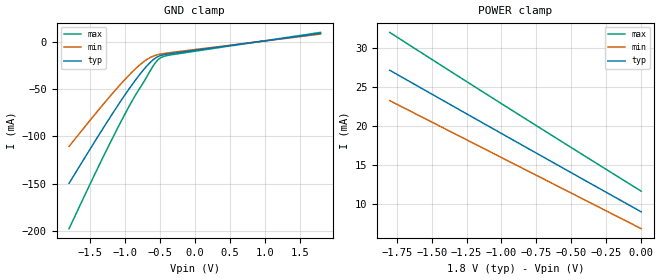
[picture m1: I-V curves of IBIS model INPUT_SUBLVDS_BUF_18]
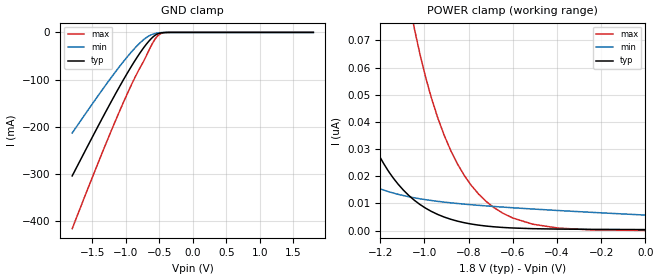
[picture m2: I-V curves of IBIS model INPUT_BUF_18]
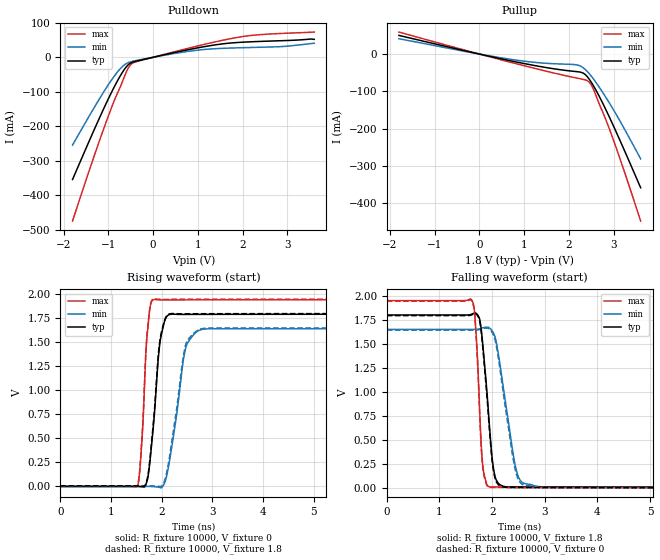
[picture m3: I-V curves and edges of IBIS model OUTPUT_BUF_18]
| TEXAS INSTRUMENTS INCORPORATED
| Digital Light Processing Group
| IBIS Model of d9696kx2sv
| P46_AUTO
| This device can be powered at the following Vccs:
|  1.8 volt Vcc
| This file provides unique models under the [Model Selector] for each Vcc.
| For operation at a specific Vcc, select the appropriate model after each
| [Model Selector] keyword.
[IBIS Ver]   3.2
[Comment char]  |_char
[File Name]   p46_auto_d9696kx2sv.ibs
[File Rev]   2.0 | f_die
[Date]   May 5, 2022
[Source]   Data created from TI-SPICE simulations at TI-DLP.
[Notes]   The following is an IBIS list for the 0.46 AUTO .
##notes##|
[Disclaimer] Property of Texas Instruments Incorporated.  Unauthorized
   reproduction and/or distribution is strictly prohibited.
   This product is protected under copyright law.
   Created  2022, (C) Copyright  2022, Texas Instruments
   Incorporated, All Rights Reserved
   UNLESS THERE IS A SIGNED, WRITTEN AGREEMENT TO THE
   CONTRARY, TEXAS INSTRUMENTS (TI) IS PROVIDING THE IBIS
   MODELS  AND WITHOUT ANY WARRANTY, EXPRESSED OR
   IMPLIED.  TI assumes no liability for:
   1) the accuracy of the IBIS models provided to your
   company;
   2) the proper functioning of these IBIS Models in your
   design or for any resulting applications; or
   3) infringement of patents, copyrights or intellectual
   property rights resulting from your use of these IBIS
   models.
   TI provides IBIS Models as a service to our customers.
   You and your company shall not distribute, sell or give
   these models to anyone else without prior written
   permission from TI.
   TI reserves the right to make changes to our products or
   to discontinue any semiconductor product or service
   without notice, and advises our customers to obtain the
   latest version of relevant information to verify, before
   placing orders, that the information being relied on is
   current.
   Please be aware that your receipt and use of the IBIS
   information provided shall serve as acceptance of these
   terms and conditions.  If you do not accept these terms,
   you should return or destroy the IBIS models and any
   other accompanying information immediately.
| Component P46_AUTO
[Component]   P46_AUTO
[Manufacturer]   Texas Instruments, Inc.
[Package]
|   typ   min   max
R_pkg   1.216   0.4680   2.140
L_pkg   6.179E-09   3.200E-09   1.320E-08
C_pkg   2.358E-12   1.500E-12   5.200E-12
|   Signal RLC
[Pin]   signal_name   model_name   R_pin   L_pin   C_pin
 A3   D_AN<0>   INPUT_SUB_LVDS_BUF   1.478   7.3E-09   2.5E-12
 B1   D_AN<1>   INPUT_SUB_LVDS_BUF   1.455   7.4E-09   2.5E-12
 C2   D_AN<2>   INPUT_SUB_LVDS_BUF   1.501   8.2E-09   2.5E-12
 F2   D_AN<3>   INPUT_SUB_LVDS_BUF   0.960   5.4E-09   2.0E-12
 H2   D_AN<4>   INPUT_SUB_LVDS_BUF   1.377   6.8E-09   2.4E-12
 K1   D_AN<5>   INPUT_SUB_LVDS_BUF   1.312   7.1E-09   2.3E-12
 K4   D_AN<6>   INPUT_SUB_LVDS_BUF   0.938   6.1E-09   2.0E-12
 K6   D_AN<7>   INPUT_SUB_LVDS_BUF   1.492   7.2E-09   2.5E-12
 A2   D_AP<0>   INPUT_SUB_LVDS_BUF   1.422   6.3E-09   2.4E-12
 C1   D_AP<1>   INPUT_SUB_LVDS_BUF   1.407   6.4E-09   2.4E-12
 D2   D_AP<2>   INPUT_SUB_LVDS_BUF   1.445   6.5E-09   2.4E-12
 E2   D_AP<3>   INPUT_SUB_LVDS_BUF   0.860   4.7E-09   2.0E-12
 G2   D_AP<4>   INPUT_SUB_LVDS_BUF   1.321   5.9E-09   2.3E-12
 K2   D_AP<5>   INPUT_SUB_LVDS_BUF   1.256   5.9E-09   2.3E-12
 K3   D_AP<6>   INPUT_SUB_LVDS_BUF   0.882   4.7E-09   2.0E-12
 K5   D_AP<7>   INPUT_SUB_LVDS_BUF   1.404   6.4E-09   2.4E-12
A22   D_BN<0>   INPUT_SUB_LVDS_BUF   1.504   6.8E-09   2.5E-12
B24   D_BN<1>   INPUT_SUB_LVDS_BUF   1.477   6.3E-09   2.5E-12
D23   D_BN<2>   INPUT_SUB_LVDS_BUF   1.154   5.3E-09   2.2E-12
F23   D_BN<3>   INPUT_SUB_LVDS_BUF   0.922   4.4E-09   1.9E-12
H23   D_BN<4>   INPUT_SUB_LVDS_BUF   1.302   6.0E-09   2.3E-12
K24   D_BN<5>   INPUT_SUB_LVDS_BUF   1.342   6.2E-09   2.4E-12
K21   D_BN<6>   INPUT_SUB_LVDS_BUF   0.894   4.9E-09   2.0E-12
K19   D_BN<7>   INPUT_SUB_LVDS_BUF   1.390   6.0E-09   2.4E-12
A23   D_BP<0>   INPUT_SUB_LVDS_BUF   1.446   6.4E-09   2.5E-12
C24   D_BP<1>   INPUT_SUB_LVDS_BUF   1.421   6.9E-09   2.4E-12
C23   D_BP<2>   INPUT_SUB_LVDS_BUF   1.096   5.8E-09   2.2E-12
E23   D_BP<3>   INPUT_SUB_LVDS_BUF   0.875   5.0E-09   1.9E-12
G23   D_BP<4>   INPUT_SUB_LVDS_BUF   1.246   5.7E-09   2.3E-12
K23   D_BP<5>   INPUT_SUB_LVDS_BUF   1.284   6.6E-09   2.3E-12
K22   D_BP<6>   INPUT_SUB_LVDS_BUF   0.839   5.1E-09   1.9E-12
K20   D_BP<7>   INPUT_SUB_LVDS_BUF   1.288   6.7E-09   2.4E-12
 J1   DCLK_AN   INPUT_SUB_LVDS_BUF   1.340   6.4E-09   2.4E-12
 H1   DCLK_AP   INPUT_SUB_LVDS_BUF   1.292   5.8E-09   2.3E-12
H24   DCLK_BN   INPUT_SUB_LVDS_BUF   1.187   5.3E-09   2.2E-12
J24   DCLK_BP   INPUT_SUB_LVDS_BUF   1.137   5.4E-09   2.2E-12
 E6   DMD_DEN_ARSTZ   INPUT_BUF   0.700   5.0E-09   2.4E-12
 C3   LS_CLK_N   INPUT_SUB_LVDS_BUF   0.468   3.2E-09   1.6E-12
 C4   LS_CLK_P   INPUT_SUB_LVDS_BUF   0.541   4.0E-09   1.5E-12
E19   LS_RDATA_A   OUTPUT_BUF   2.041   12.8E-09   5.0E-12
F19   LS_RDATA_B   OUTPUT_BUF   2.140   13.2E-09   5.2E-12
 C5   LS_WDATA_N   INPUT_SUB_LVDS_BUF   0.694   3.8E-09   1.8E-12
 C6   LS_WDATA_P   INPUT_SUB_LVDS_BUF   0.741   4.4E-09   1.8E-12
C18   MBRST<0>   NC
C17   MBRST<1>   NC
D18   MBRST<6>   NC
D17   MBRST<7>   NC
 F6   TEMP_N   NC
 G6   TEMP_P   NC
E18   TP0   NC
E17   TP1   NC
E16   TP2   NC
 A4   VBIAS   POWER
A21   VBIAS   POWER
A24   VSS   GND
 B2   VSS   GND
 B3   VOFFSET   POWER
 B4   VOFFSET   POWER
 B5   VSS   GND
 B6   VRESET   POWER
B19   VRESET   POWER
B20   VSS   GND
B21   VOFFSET   POWER
B22   VOFFSET   POWER
B23   VSS   GND
C19   VSS   GND
C20   VDD   POWER
C21   VSS   GND
C22   VSS   GND
 D3   VSS   GND
 D4   VDD   POWER
 D5   VSS   GND
 D6   VSS   GND
D19   VDD   POWER
D20   VSS   GND
D21   VDD   POWER
D22   VSS   GND
 E3   VDD   POWER
 E4   VSS   GND
 E5   VDDI   POWER
E20   VDDI   POWER
E21   VSS   GND
E22   VDD   POWER
 F3   VSS   GND
 F4   VDD   POWER
 F5   VDDI   POWER
F20   VDDI   POWER
F21   VSS   GND
F22   VSS   GND
 G3   VDD   POWER
 G4   VSS   GND
 G5   VDDI   POWER
G19   VSS   GND
G20   VDDI   POWER
G21   VDD   POWER
G22   VSS   GND
 H3   VSS   GND
 H4   VSS   GND
 H5   VDDI   POWER
 H6   VSS   GND
H19   VSS   GND
H20   VDDI   POWER
H21   VSS   GND
H22   VDD   POWER
 J2   VSS   GND
 J3   VDD   POWER
 J4   VOFFSET   POWER
 J5   VSS   GND
 J6   VDD   POWER
J19   VDD   POWER
J20   VSS   GND
J21   VOFFSET   POWER
J22   VSS   GND
J23   VSS   GND
| NOTE:  The [Diff Pin] section may get flagged by early versions of the
|   ibischk program
[Diff Pin]  inv_pin   vdiff   tdelay_typ
A2   A3   200mv   NA
C1   B1   200mv   NA
D2   C2   200mv   NA
E2   F2   200mv   NA
G2   H2   200mv   NA
K2   K1   200mv   NA
K3   K4   200mv   NA
K5   K6   200mv   NA
A23   A22   200mv   NA
C24   B24   200mv   NA
C23   D23   200mv   NA
E23   F23   200mv   NA
G23   H23   200mv   NA
K23   K24   200mv   NA
K22   K21   200mv   NA
K20   K19   200mv   NA
H1   J1   200mv   NA
J24   H24   200mv   NA
C4   C3   200mv   NA
C6   C5   200mv   NA
| Model INPUT_SUB_LVDS_BUF
[Model Selector]   INPUT_SUB_LVDS_BUF
INPUT_SUBLVDS_BUF_18   1.8 volt Vcc
| Model INPUT_BUF
[Model Selector]   INPUT_BUF
INPUT_BUF_18   1.8 volt Vcc
| Model OUTPUT_BUF
[Model Selector]   OUTPUT_BUF
OUTPUT_BUF_18   1.8 volt Vcc
| Models and submodels in the file (3): INPUT_SUBLVDS_BUF_18 (Input), INPUT_BUF_18 (Input), OUTPUT_BUF_18 (Output)
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[Model]   INPUT_SUBLVDS_BUF_18
Model_type  Input
Vinl=0.80
Vinh=1.00
| variable   typ   min   max
C_comp   0.69pF   0.66pF   0.72pF
[Temperature Range]   25   85   -40
[Voltage range]   1.8   1.65   1.95
[GND Clamp]
| INPUT_SUBLVDS_BUF_18
|   Voltage   I(typ)   I(min)   I(max)
-1.8V     -149.7mA   -110.7mA   -197.8mA
-1.29V    -88.84mA   -64.29mA   -118.6mA
-1.095V   -66.55mA   -47.56mA   -89.83mA
-930mV    -48.67mA   -34.42mA   -66.87mA
-790mV    -34.7mA    -24.56mA   -49.3mA
-680mV    -25.03mA   -18.39mA   -35.98mA
-580mV    -18.08mA   -14.73mA   -23.73mA
-510mV    -15.09mA   -13.26mA   -17.94mA
-450mV    -13.75mA   -12.43mA   -15.53mA
-355mV    -12.57mA   -11.45mA   -13.96mA
1.8V      8.993mA    8.203mA    9.976mA
[POWER Clamp]
| INPUT_SUBLVDS_BUF_18
|   Voltage   I(typ)   I(min)   I(max)
-1.8V     27.16mA    23.26mA    32.02mA
-1.37V    22.79mA    19.34mA    27.08mA
-920mV    18.24mA    15.23mA    21.97mA
-16.28fV  8.993mA    6.835mA    11.65mA
[Model]   INPUT_BUF_18
Model_type  Input
Vinl=0.54
Vinh=1.26
| variable   typ   min   max
C_comp   0.51pF   0.44pF   0.58pF
[Temperature Range]   25   85   -40
[Voltage range]   1.8   1.65   1.95
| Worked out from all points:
|   GND clamp passes 1 mA (typ) near -0.47 V on its own axis
[GND Clamp]
| INPUT_BUF_18
|   Voltage   I(typ)   I(min)   I(max)
-1.8V     -304mA     -213.1mA   -415.8mA
-1.52V    -227.4mA   -155.6mA   -314.4mA
-1.29V    -165.7mA   -109.6mA   -233.4mA
-1.095V   -115.3mA   -72.59mA   -167.6mA
-930mV    -75.06mA   -43.75mA   -115.2mA
-790mV    -43.93mA   -22.51mA   -75.55mA
-680mV    -22.72mA   -9.755mA   -45.56mA
-580mV    -7.998mA   -2.996mA   -17.96mA
-510mV    -2.379mA   -972.8uA   -5.564mA
-450mV    -592.5uA   -304.6uA   -1.296mA
-355mV    -35.15uA   -32.8uA    -61.22uA
1.8V      384pA      6.33nA     42.47pA
[POWER Clamp]
| INPUT_BUF_18
|   Voltage   I(typ)   I(min)   I(max)
-1.8V     438.6nA    109.4nA    1.836uA
-1.7V     293.4nA    73.99nA    1.296uA
-1.565V   164.4nA    44.27nA    784.1nA
-1.4V     75.97nA    25.31nA    401.7nA
-1.255V   36.21nA    17.25nA    210.8nA
-1.155V   20.97nA    14.17nA    130.5nA
-1.045V   11.14nA    12.07nA    74.21nA
-970mV    7.14nA     11.1nA     49.29nA
-880mV    4.163nA    10.23nA    29.33nA
-685mV    1.408nA    8.888nA    8.453nA
-395mV    567.5pA    7.406nA    949.3pA
-16.28fV  384pA      5.724nA    60.79pA
[Model]   OUTPUT_BUF_18
Model_type  Output
Vref =   0
Rref =   10000
Cref =   10p
Vmeas =   1.2
| variable   typ   min   max
C_comp   0.65pF   0.45pF   1.15pF
| C_pullup   0.66pF   0.45pF   1.15pF
| C_pulldown   0.63pF   0.50pF   1.03pF
[Temperature Range]   25   85   -40
[Voltage range]   1.8   1.65   1.95
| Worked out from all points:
|   slope of the pulldown table from 0 to 0.27 V, typ, clamps not added: 34.3 ohm
|   slope of the pullup table from 0 to 0.27 V, typ, clamps not added: 37.6 ohm
|   rising waveform, R_fixture 10000, V_fixture 0: 20-80 % time 164ps typ, 253ps min, 111ps max; typ from 0 V to 1.79 V
|   falling waveform, R_fixture 10000, V_fixture 1.8: 20-80 % time 159ps typ, 266ps min, 98.4ps max; typ from 1.8 V to 0.006 V
|   rising waveform, R_fixture 10000, V_fixture 1.8: 20-80 % time 164ps typ, 256ps min, 110ps max; typ from 0.006 V to 1.8 V
|   falling waveform, R_fixture 10000, V_fixture 0: 20-80 % time 159ps typ, 263ps min, 98.5ps max; typ from 1.79 V to 0 V
[Pulldown]
| OUTPUT_BUF_18
|   Voltage   I(typ)   I(min)   I(max)
-1.8V     -354.2mA   -254.4mA   -474.4mA
-1.265V   -195mA     -134.5mA   -266.6mA
-895mV    -92.67mA   -59.47mA   -134.6mA
-755mV    -58.61mA   -36.11mA   -91.94mA
-645mV    -35.65mA   -22.4mA    -56.96mA
-555mV    -21.67mA   -15.53mA   -31.37mA
-480mV    -15.3mA    -12.24mA   -19.11mA
-345mV    -10.18mA   -8.457mA   -11.8mA
875mV     24.33mA    18.74mA    29.04mA
1.865V    42.67mA    27.28mA    57.21mA
2.905V    48.22mA    31.33mA    69.32mA
3.6V      52.02mA    40.86mA    73.18mA
[Pullup]
| OUTPUT_BUF_18
|   Voltage   I(typ)   I(min)   I(max)
-1.8V     49.99mA    41.08mA    59.07mA
730mV     -18.9mA    -14.55mA   -23.06mA
1.36V     -33.47mA   -23.55mA   -42.08mA
2.165V    -46.93mA   -28.87mA   -64.13mA
2.32V     -51.32mA   -37.02mA   -67.96mA
2.435V    -64.68mA   -50.22mA   -73.6mA
2.49V     -74.19mA   -58.09mA   -81.45mA
2.545V    -84.87mA   -66.63mA   -94.28mA
2.7V      -119.1mA   -93.19mA   -140.9mA
2.895V    -167.2mA   -129.8mA   -198.5mA
3.195V    -246.7mA   -191.5mA   -300.4mA
3.6V      -358.2mA   -280.8mA   -447.3mA
[Ramp]
| OUTPUT_BUF_18
| variable   typ   min   max
dV/dt_r   1.08/1.67E-10   0.99/2.58E-10   1.17/1.11E-10
dV/dt_f   1.09/1.62E-10   1.00/2.72E-10   1.18/1.01E-10
R_load = 10000
[Rising Waveform]
| OUTPUT_BUF_18
R_fixture =   10000
C_fixture =   0
L_fixture =   0
V_fixture =   0
V_fixture_min = 0
V_fixture_max = 0
|   Time   V(typ)   V(min)   V(max)
0s        2.935nV    32.33nV    304.2pV
1.525ns   12.81uV    20.21uV    4.084mV
1.615ns   -3.833mV   105uV      533.5mV
1.71ns    58.13mV    123.1uV    1.568V
1.855ns   750.8mV    -2.782mV   1.947V
1.955ns   1.458V     -9.919mV   1.942V
2.08ns    1.753V     73.73mV    1.941V
2.47ns    1.791V     1.436V     1.942V
2.825ns   1.792V     1.638V     1.943V
24.99ns   1.793V     1.642V     1.944V
[Falling Waveform]
| OUTPUT_BUF_18
R_fixture =   10000
C_fixture =   0
L_fixture =   0
V_fixture =   1.8
V_fixture_min = 1.65
V_fixture_max = 1.95
|   Time   V(typ)   V(min)   V(max)
0s        1.8V       1.65V      1.95V
1.62ns    1.81V      1.65V      1.949V
1.69ns    1.819V     1.651V     1.653V
1.76ns    1.764V     1.656V     844.3mV
1.82ns    1.507V     1.667V     244.5mV
1.955ns   601.1mV    1.662V     9.6mV
2.08ns    79.45mV    1.512V     9.328mV
2.475ns   9.39mV     152mV      8.293mV
2.885ns   8.404mV    13.17mV    7.567mV
24.99ns   6.04mV     6.675mV    5.66mV
[Rising Waveform]
| OUTPUT_BUF_18
R_fixture =   10000
C_fixture =   0
L_fixture =   0
V_fixture =   1.8
V_fixture_min = 1.65
V_fixture_max = 1.95
|   Time   V(typ)   V(min)   V(max)
0s        6.039mV    6.675mV    5.66mV
1.525ns   6.058mV    6.695mV    10.55mV
1.61ns    2.738mV    6.771mV    514.5mV
1.71ns    72.65mV    6.795mV    1.588V
1.855ns   789.8mV    4.171mV    1.952V
1.955ns   1.486V     187.2uV    1.948V
2.08ns    1.761V     104.7mV    1.948V
2.465ns   1.798V     1.459V     1.948V
2.825ns   1.798V     1.646V     1.949V
24.99ns   1.8V       1.65V      1.95V
[Falling Waveform]
| OUTPUT_BUF_18
R_fixture =   10000
C_fixture =   0
L_fixture =   0
V_fixture =   0
V_fixture_min = 0
V_fixture_max = 0
|   Time   V(typ)   V(min)   V(max)
0s        1.793V     1.642V     1.944V
1.62ns    1.803V     1.642V     1.942V
1.69ns    1.811V     1.643V     1.63V
1.76ns    1.748V     1.648V     814.7mV
1.815ns   1.504V     1.657V     253.2mV
1.955ns   560.3mV    1.649V     4.112mV
2.075ns   66.14mV    1.49V      3.651mV
2.465ns   3.348mV    135.5mV    2.653mV
2.86ns    2.404mV    7.718mV    1.943mV
24.99ns   6.498nV    37.43nV    3.212nV
